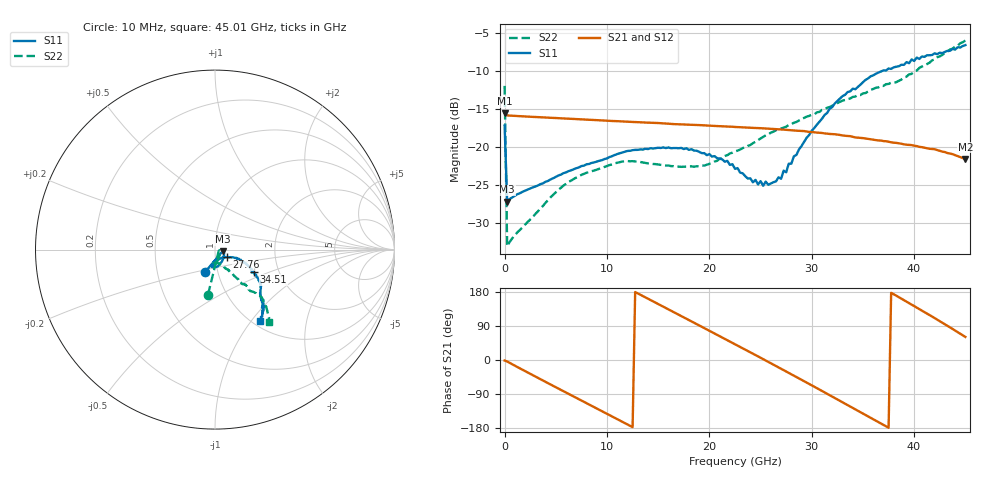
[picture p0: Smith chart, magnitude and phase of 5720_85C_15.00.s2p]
! Device:  ADRF5720
! Description: 0.5dB LSB GaAs MMIC 6-bit Digital Attenuator
! Frequency:  0.000009 -  40 GHz
! Ports:
!	RF1	= Port 1
!	RF2	= Port 2
! Vdd:  3.3 Volt
! Vss:  -3.3 Volt
! Control:  0/3.3 Volt
! State:  15.00 dB attenuation
! Data:  The device was measured using G-S-G Probes on a matrix board.
!  Data was collected using an calibrated 4 port network analyzer.
!  The reference plane for this measurement is at the launchers.
! Note:  Analog Devices supplies this data as a sample of measured data
!  for this product.  Your particular data for this product may vary.
!  Data was taken at 85 degrees C.
!  Analog Devices reserves the right to change this data at anytime.
# GHZ S DB R 45.0
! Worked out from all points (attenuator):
!   181 points, 10 MHz to 45.01 GHz, reference 45 ohm
!   highest |S21| = -15.54 dB at 10 MHz (marker M1); lowest = -21.6 dB at 45.01 GHz (marker M2)
!   lowest |S11| = -27.2 dB at 260 MHz (marker M3), VSWR 1.09, Z = 49 - j0.854 ohm
!   |S11| at or under -10 dB: start of sweep to 36.82 GHz
!   |S22| runs from -33.1 to -5.9 dB; largest |S21 - S12| = 0.00086
!   S11 on the Smith chart (normalised r, x): 10 MHz: 0.87, -0.22; 27.76 GHz: 1.14, -0.10; 34.51 GHz: 1.49, -0.39; 45.01 GHz: 1.08, -1.10
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0.01  -17.16 -114.0  -15.54 -1.4  -15.52 -1.4  -11.93 -98.8
0.26  -27.19 -11.5  -15.83 -4.0  -15.82 -3.9  -33.07 -21.6
4.26  -24.46 -35.6  -16.12 -61.3  -16.10 -61.2  -26.99 -58.0
7.76  -22.45 -58.8  -16.36 -110.5  -16.35 -110.5  -23.53 -80.1
11.51  -20.71 -78.3  -16.62 -163.1  -16.61 -163.0  -21.91 -94.0
15.26  -20.12 -92.2  -16.85 144.1  -16.84 144.2  -22.35 -96.5
19.51  -20.80 -100.2  -17.14 84.2  -17.13 84.4  -22.44 -79.8
22.76  -22.77 -94.6  -17.36 38.1  -17.35 38.3  -20.47 -66.3
24.26  -24.65 -85.4  -17.47 16.7  -17.46 16.9  -19.49 -62.6
25.01  -24.49 -75.2  -17.51 5.9  -17.50 6.2  -18.87 -62.1
25.26  -25.11 -73.7  -17.53 2.3  -17.51 2.6  -18.65 -60.9
27.01  -24.18 -43.5  -17.67 -23.1  -17.65 -22.8  -17.56 -57.1
27.51  -23.32 -37.0  -17.73 -30.4  -17.72 -30.1  -17.31 -56.4
27.76  -22.19 -33.0  -17.75 -34.0  -17.74 -33.7  -17.09 -57.0
28.01  -22.20 -32.6  -17.79 -37.7  -17.77 -37.4  -16.98 -56.3
30.26  -17.48 -23.0  -18.05 -70.6  -18.03 -70.3  -15.69 -54.6
33.01  -13.28 -26.6  -18.47 -111.5  -18.45 -111.2  -13.88 -52.7
34.51  -12.07 -29.9  -18.76 -133.6  -18.74 -133.3  -13.12 -52.7
35.76  -10.67 -34.3  -18.96 -152.5  -18.95 -152.2  -12.45 -52.0
37.76  -9.69 -39.3  -19.37 177.2  -19.35 177.6  -11.52 -49.1
41.51  -7.89 -48.9  -20.23 118.8  -20.20 119.2  -8.87 -45.6
45.01  -6.55 -58.0  -21.57 60.9  -21.55 61.2  -5.94 -53.3
